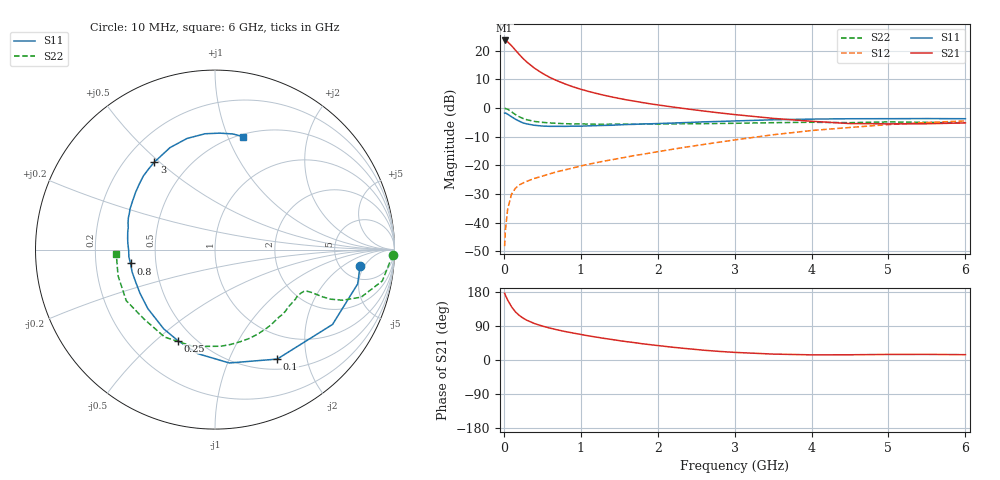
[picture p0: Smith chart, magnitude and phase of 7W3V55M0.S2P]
! Infineon Technologies  Discrete & RF Semiconductors
! BFS17W
! Si NPN RF Bipolar Junction Transistor in SOT323
! VCE = 3.5 V  IC = 5 mA
! Common Emitter S-Parameters:  August  1999
# GHz  S  MA  R  50
!  f  S11  S21  S12  S22
! GHz  MAG  ANG  MAG  ANG  MAG  ANG  MAG  ANG
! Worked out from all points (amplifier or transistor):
!   36 points, 10 MHz to 6 GHz, reference 50 ohm
!   highest |S21| = 23.5 dB at 10 MHz (marker M1)
!   |S21| within 3 dB of that: start of sweep to 138.4 MHz
!   unconditionally stable (mu >= 1): 554.4 MHz to 2.787 GHz; 4.306 GHz to end of sweep
!   at 250 MHz: K = 0.59, MSG = 21.7 dB, |S12| = -26.2 dB
!   at 1.4 GHz: K = 1.25, MAG = 7.9 dB, |S12| = -18.1 dB
!   at 6 GHz: K = 1.08, MAG = -2.1 dB, |S12| = -4.5 dB
!   S11 on the Smith chart (normalised r, x): 10 MHz: 7.42, -4.10; 100 MHz: 0.64, -1.53; 250 MHz: 0.41, -0.59; 800 MHz: 0.36, -0.07; 3 GHz: 0.32, +0.48; 6 GHz: 0.52, +1.14
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0.01  0.8133 -6.6  14.98 176.0  0.0039 87.6  0.9941 -1.8
0.02  0.8177 -13.5  14.94 171.0  0.0073 87.9  0.9749 -4.4
0.05  0.7763 -32.5  14.14 158.1  0.0174 74.1  0.9485 -10.6
0.1  0.7015 -60.4  12.14 140.5  0.0313 62.5  0.8566 -18.0
0.15  0.6367 -82.8  10.18 127.1  0.0398 54.2  0.766 -21.6
0.2  0.5879 -99.3  8.546 117.8  0.0455 51.6  0.7015 -23.2
0.25  0.5475 -112.3  7.256 110.5  0.0491 48.4  0.6538 -23.7
0.3  0.5259 -122.9  6.282 104.8  0.0528 48.6  0.6223 -23.8
0.4  0.4981 -138.7  4.913 96.1  0.0592 48.5  0.5812 -24.0
0.5  0.4836 -149.8  4.02 89.6  0.0648 50.3  0.5603 -24.4
0.6  0.4774 -157.9  3.386 84.1  0.0712 52.5  0.547 -25.2
0.8  0.477 -170.7  2.605 75.0  0.0836 55.7  0.531 -28.2
0.9  0.4816 -175.2  2.33 71.2  0.0901 57.1  0.5267 -29.8
1.1  0.4868 175.9  1.941 63.7  0.1044 59.6  0.5229 -34.0
1.3  0.4958 168.7  1.667 57.2  0.1183 61.1  0.5189 -38.7
1.6  0.5147 159.6  1.378 48.3  0.1395 63.1  0.5186 -46.1
2.2  0.5456 144.1  1.035 33.6  0.1911 65.8  0.5274 -62.8
3  0.593 124.8  0.766 20.1  0.2767 64.3  0.5394 -86.6
3.5  0.6211 113.8  0.658 15.6  0.3408 60.7  0.5532 -102.6
4.5  0.6478 94.9  0.534 13.8  0.4565 48.8  0.5532 -135.7
5.5  0.652 81.2  0.53 14.8  0.5552 36.2  0.5595 -164.9
6  0.6485 76.0  0.548 14.1  0.5936 30.0  0.5507 -177.7
